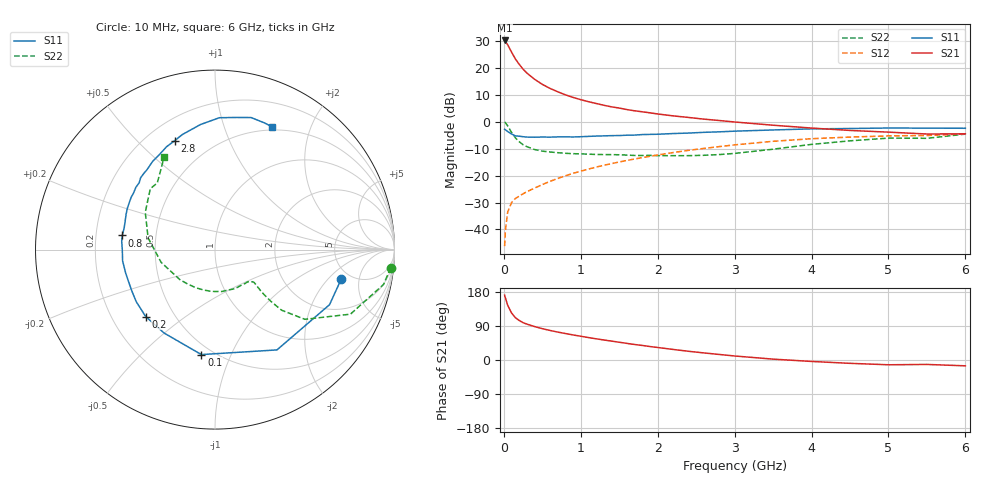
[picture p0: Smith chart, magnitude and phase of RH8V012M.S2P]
! SIEMENS Small Signal Semiconductors
! BFR106
! Si NPN RF Bipolar Junction Transistor in SOT23
! VCE = 8 V  IC = 12 mA
! Common Emitter S-Parameters:  August  1996
# GHz  S  MA  R  50
!  f  S11  S21  S12  S22
! GHz  MAG  ANG  MAG  ANG  MAG  ANG  MAG  ANG
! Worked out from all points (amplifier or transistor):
!   36 points, 10 MHz to 6 GHz, reference 50 ohm
!   highest |S21| = 30.1 dB at 10 MHz (marker M1)
!   |S21| within 3 dB of that: start of sweep to 75.74 MHz
!   unconditionally stable (mu >= 1): 462.3 MHz to 2.024 GHz; 5.479 GHz to 5.698 GHz
!   at 250 MHz: K = 0.75, MSG = 23.1 dB, |S12| = -26.8 dB
!   at 1.4 GHz: K = 1.08, MAG = 8.8 dB, |S12| = -15.6 dB
!   at 6 GHz: K = 1.00, MSG = 0.0 dB, |S12| = -4.6 dB
!   S11 on the Smith chart (normalised r, x): 10 MHz: 4.19, -2.85; 100 MHz: 0.43, -0.78; 200 MHz: 0.35, -0.36; 800 MHz: 0.32, +0.07; 2.8 GHz: 0.31, +0.65; 6 GHz: 0.46, +1.47
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0.01  0.7227 -13.0  32.09 171.2  0.0049 86.7  0.9842 -5.9
0.02  0.7081 -25.7  31.14 164.2  0.0095 77.5  0.9589 -11.7
0.05  0.6569 -58.3  26.66 144.5  0.021 64.2  0.8358 -25.5
0.1  0.5898 -97.4  19.53 124.2  0.0316 54.1  0.6338 -37.8
0.15  0.5446 -121.4  14.57 111.6  0.0375 49.9  0.5017 -42.3
0.2  0.5369 -136.0  11.56 104.3  0.0416 49.8  0.4251 -42.8
0.25  0.5261 -146.5  9.422 98.5  0.0459 50.6  0.373 -42.5
0.3  0.5174 -153.8  7.971 94.6  0.0503 52.9  0.3437 -42.1
0.4  0.5146 -165.1  6.105 88.2  0.0586 55.9  0.3039 -40.7
0.5  0.5186 -173.0  4.919 82.7  0.068 58.7  0.2837 -40.0
0.6  0.5164 -179.6  4.144 78.0  0.0782 60.8  0.2739 -40.8
0.8  0.5227 171.3  3.149 69.9  0.099 63.2  0.259 -43.7
0.9  0.5202 166.5  2.818 66.1  0.11 63.8  0.2547 -45.4
1.1  0.533 158.3  2.348 59.2  0.1318 64.3  0.2497 -51.2
1.3  0.5446 151.3  2.014 52.8  0.1551 63.8  0.2451 -57.0
1.6  0.5611 141.8  1.676 43.8  0.1905 62.3  0.2399 -67.9
2.2  0.6017 125.3  1.281 27.9  0.2671 56.7  0.2338 -94.5
2.8  0.6471 110.3  1.05 14.6  0.3444 48.8  0.2452 -128.8
3.5  0.7016 96.6  0.859 2.3  0.4323 38.0  0.3085 -166.7
4.5  0.7458 80.8  0.687 -8.8  0.5178 20.9  0.4408 151.8
5.5  0.7578 68.8  0.59 -11.7  0.5538 9.0  0.491 130.9
6  0.7542 64.9  0.595 -15.4  0.592 1.0  0.5873 118.9
